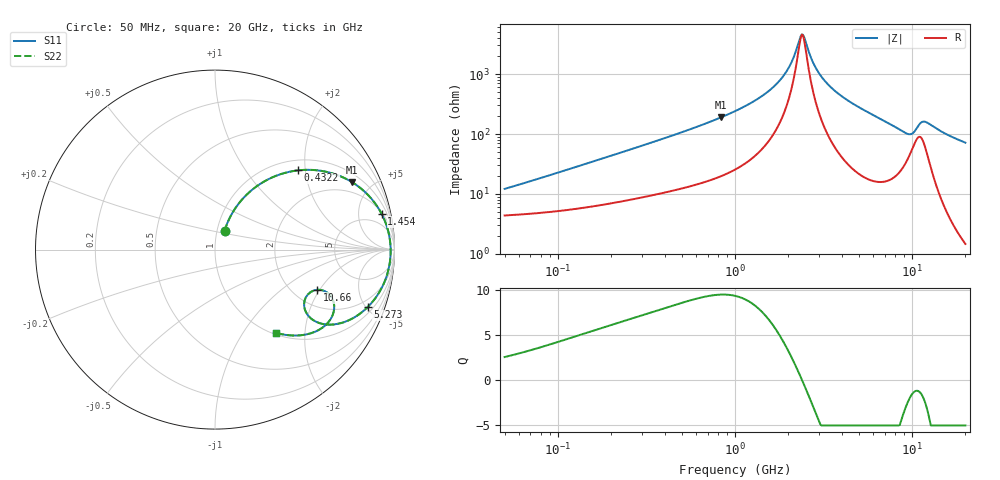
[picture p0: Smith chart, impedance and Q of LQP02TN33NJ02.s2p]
!Murata Part Number: LQP02TN33NJ02
!These Parameters are Measured in Series Mode Connection
!  o--[Z]--o
!Port1  Port2
!  o-------o
!Freq. Start=50[MHz] Stop=20[GHz], 401[Steps]
# Hz S RI R 50
!Freq.(Hz) S11(Real) S11(Imag) S21(Real) S21(Imag) S12(Real) S12(Imag) S22(Real) S22(Imag)
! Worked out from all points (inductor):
!   401 points, 50 MHz to 20 GHz, reference 50 ohm
!   read as one part in series: L = 35.5 nH near 60.75 MHz
!   highest Q = 9.52 at 835.5 MHz (marker M1), where L = 36 nH
!   self-resonance near 2.384 GHz
!   S11 on the Smith chart (normalised r, x): 50 MHz: 1.09, +0.23; 432.2 MHz: 1.22, +1.83; 1.454 GHz: 2.21, +8.94; 5.273 GHz: 1.39, -5.12; 10.66 GHz: 2.66, -1.91; 20 GHz: 1.03, -1.43
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5e7  0.0532 0.103  0.9468 -0.103  0.9468 -0.103  0.0532 0.103
1.364002e8  0.1244 0.2463  0.8756 -0.2463  0.8756 -0.2463  0.1244 0.2463
3.721004e8  0.3984 0.4298  0.6016 -0.4298  0.6016 -0.4298  0.3984 0.4298
4.322267e8  0.4632 0.4415  0.5368 -0.4415  0.5368 -0.4415  0.4632 0.4415
8.354841e8  0.7606 0.3774  0.2394 -0.3774  0.2394 -0.3774  0.7606 0.3774
1e9  0.8279 0.328  0.1721 -0.328  0.1721 -0.328  0.8279 0.328
1.454215e9  0.9289 0.1981  0.0711 -0.1981  0.0711 -0.1981  0.9289 0.1981
1.932977e9  0.9688 0.0868  0.0312 -0.0868  0.0312 -0.0868  0.9688 0.0868
2.083303e9  0.9742 0.0567  0.0258 -0.0567  0.0258 -0.0567  0.9742 0.0567
2.383959e9  0.9787 0.00195  0.0213 -0.00195  0.0213 -0.00195  0.9787 0.00195
2.456456e9  0.9788 -0.0103  0.0212 0.0103  0.0212 0.0103  0.9788 -0.0103
2.728004e9  0.9764 -0.0534  0.0236 0.0534  0.0236 0.0534  0.9764 -0.0534
3.029571e9  0.9698 -0.0967  0.0302 0.0967  0.0302 0.0967  0.9698 -0.0967
3.466789e9  0.9547 -0.1526  0.0453 0.1526  0.0453 0.1526  0.9547 -0.1526
5.273168e9  0.8501 -0.3208  0.1499 0.3208  0.1499 0.3208  0.8501 -0.3208
7.442007e9  0.6709 -0.4158  0.3291 0.4158  0.3291 0.4158  0.6709 -0.4158
9.457416e9  0.5007 -0.3337  0.4993 0.3337  0.4993 0.3337  0.5007 -0.3337
1.066139e10  0.5708 -0.2236  0.4292 0.2236  0.4292 0.2236  0.5708 -0.2236
1.149051e10  0.6538 -0.2733  0.3462 0.2733  0.3462 0.2733  0.6538 -0.2733
1.238412e10  0.6565 -0.362  0.3435 0.362  0.3435 0.362  0.6565 -0.362
1.482269e10  0.5348 -0.4659  0.4652 0.4659  0.4652 0.4659  0.5348 -0.4659
2e10  0.3425 -0.4644  0.6575 0.4644  0.6575 0.4644  0.3425 -0.4644
